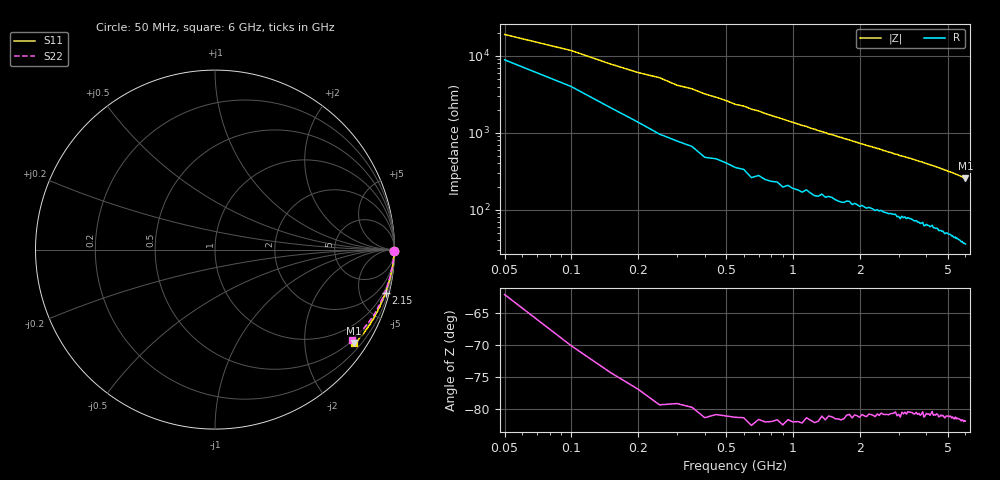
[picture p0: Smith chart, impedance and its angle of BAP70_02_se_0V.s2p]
!	Created	by	janssen	on	Thu	Dec	12	13:21:17	MET	2002
#	HZ	S	MA	R	50
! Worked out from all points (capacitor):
!   120 points, 50 MHz to 6 GHz, reference 50 ohm
!   read as one part in series: C = 144 fF near 50 MHz
!   lowest |Z| = 255 ohm at 6 GHz (marker M1)
!   S11 on the Smith chart (normalised r, x): 50 MHz: open; 2.15 GHz: 0.66, -7.98; 6 GHz: 0.39, -3.23
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5e7  0.9977 -0.5  0.00525 61.6  0.005712 62.2  0.9978 -0.4
1e8  0.9974 -0.9  0.008499 69.3  0.008349 63.3  0.9974 -0.8
1.5e8  0.997 -1.2  0.01267 73.1  0.01199 73.9  0.997 -1.1
2e8  0.9972 -1.5  0.01639 75.4  0.01602 76.2  0.9969 -1.5
2.5e8  0.9963 -1.9  0.01911 77.5  0.01935 77.4  0.9963 -1.9
3e8  0.9971 -2.2  0.02395 76.9  0.02338 78.4  0.9966 -2.2
3.5e8  0.9967 -2.6  0.02662 77.1  0.02727 77.0  0.9959 -2.6
4e8  0.9952 -3.0  0.03102 78.4  0.03041 77.5  0.9951 -3.0
4.5e8  0.9966 -3.3  0.03424 77.6  0.0343 77.8  0.9946 -3.3
5.5e8  0.995 -4.1  0.04237 77.3  0.04122 78.0  0.9942 -4.0
6e8  0.9962 -4.4  0.04455 77.0  0.04537 77.9  0.9933 -4.4
6.5e8  0.9945 -4.7  0.04892 77.9  0.04779 77.1  0.9936 -4.7
7e8  0.9945 -5.1  0.05154 76.6  0.0524 76.3  0.9921 -5.1
8e8  0.9932 -5.8  0.05903 76.2  0.05877 76.1  0.9918 -5.8
1.05e9  0.9915 -7.5  0.07557 74.5  0.07605 75.2  0.9885 -7.5
1.45e9  0.9868 -10.1  0.1014 71.1  0.1008 71.6  0.9834 -10.0
2.05e9  0.9804 -13.6  0.135 67.3  0.1356 67.9  0.9778 -13.6
2.15e9  0.9799 -14.2  0.1406 67.1  0.1428 67.4  0.9765 -14.1
3.05e9  0.973 -19.1  0.1884 62.2  0.1914 61.8  0.9654 -19.0
4.05e9  0.9637 -23.7  0.2354 57.2  0.2394 56.9  0.954 -23.5
5.05e9  0.9511 -28.7  0.2865 52.6  0.291 51.4  0.9361 -28.4
6e9  0.9356 -34.0  0.339 48.1  0.3408 46.7  0.9125 -33.4
